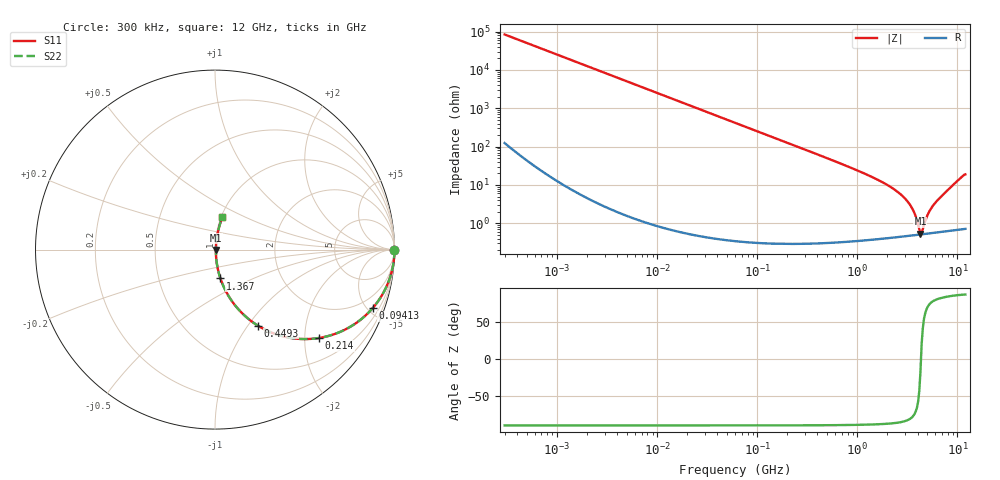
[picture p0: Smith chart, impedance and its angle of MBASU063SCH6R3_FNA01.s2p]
! MBASU063SCH6R3_FNA01  S-PARAMETER MODEL  ( General Type )
! Model Generated by TAIYO YUDEN Corporation (http://www.ty-top.com)
! Version 1.0
! TAIYO YUDEN Control No. 130801
! Copyright(c) 2013 TAIYO YUDEN CO.,LTD. All Rights Reserved.
! Product Description (link to TY-COMPAS)
! https://ds.yuden.co.jp/TYCOMPAS/or/detail?pn=MBASU063SCH6R3DFNA01&u=M
! Products Name : Multilayer Ceramic Capacitors
! Characteristics :
!  Capacitance : 6.3 pF , Rated Voltage : 50V , TCC : CH / C0H
!  Case Size : 0.6 x 0.3 / 0.024 x 0.012 [mm/inch] , Thickness : 0.3 / 0.012 [mm/inch]
!  (Conditions: Temperature = 25 degC , DC Bias Current/Voltage = 0A / 0V)
! External Node Assignments :
!  1  o---| |---o  2
! GND o---------o GND
! Frequency Range : 0.3MHz  -  12000MHz  [ 401 STEP ]
# MHz S RI R 50
! Freq[MHz].  S11 Real  S11 Imag  S21 Real  S21 Imag  S12 Real  S12 Imag  S22 Real  S22 Imag
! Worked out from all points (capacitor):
!   401 points, 300 kHz to 12 GHz, reference 50 ohm
!   read as one part in series: C = 6.3 pF near 316.3 kHz
!   lowest |Z| = 533 mohm at 4.271 GHz (marker M1)
!   series resonance near 4.322 GHz, so ESL is about 220 pH
!   S11 on the Smith chart (normalised r, x): 300 kHz: open; 94.13 MHz: 1.01, -5.37; 214 MHz: 1.01, -2.36; 449.3 MHz: 1.01, -1.11; 1.367 GHz: 1.01, -0.33; 12 GHz: 1.01, +0.38
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0.3  1 -0.00119  3.16e-06 0.00119  3.16e-06 0.00119  1 -0.00119
1.769972  0.9999 -0.007  5.17e-05 0.007  5.17e-05 0.007  0.9999 -0.007
10.44266  0.9983 -0.0413  0.00172 0.0413  0.00172 0.0413  0.9983 -0.0413
27.82928  0.988 -0.1088  0.012 0.1088  0.012 0.1088  0.988 -0.1088
60  0.9465 -0.2247  0.0535 0.2247  0.0535 0.2247  0.9465 -0.2247
94.13233  0.8778 -0.327  0.1222 0.327  0.1222 0.327  0.8778 -0.327
213.9924  0.581 -0.4922  0.419 0.4922  0.419 0.4922  0.581 -0.4922
353.9943  0.3352 -0.47  0.6648 0.47  0.6648 0.47  0.3352 -0.47
449.3064  0.2376 -0.4229  0.7624 0.4229  0.7624 0.4229  0.2376 -0.4229
743.2595  0.1005 -0.2958  0.8995 0.2958  0.8995 0.2958  0.1005 -0.2958
1366.97  0.0304 -0.1608  0.9696 0.1608  0.9696 0.1608  0.0304 -0.1608
2088.533  0.0126 -0.0913  0.9874 0.0913  0.9874 0.0913  0.0126 -0.0913
2722.03  0.00754 -0.0555  0.9925 0.0555  0.9925 0.0555  0.00754 -0.0555
3276.641  0.00576 -0.0326  0.9942 0.0326  0.9942 0.0326  0.00576 -0.0326
3642.919  0.00525 -0.0201  0.9948 0.0201  0.9948 0.0201  0.00525 -0.0201
4158.869  0.00507 -0.00465  0.9949 0.00465  0.9949 0.00465  0.00507 -0.00465
4270.516  0.00509 -0.00151  0.9949 0.00151  0.9949 0.00151  0.00509 -0.00151
4502.883  0.00519 0.00453  0.9948 -0.00453  0.9948 -0.00453  0.00519 0.00453
5140.631  0.0057 0.0175  0.9943 -0.0175  0.9943 -0.0175  0.0057 0.0175
5868.704  0.00659 0.0309  0.9934 -0.0309  0.9934 -0.0309  0.00659 0.0309
9708.23  0.0204 0.1159  0.9796 -0.1159  0.9796 -0.1159  0.0204 0.1159
12000  0.0409 0.18  0.9591 -0.18  0.9591 -0.18  0.0409 0.18
